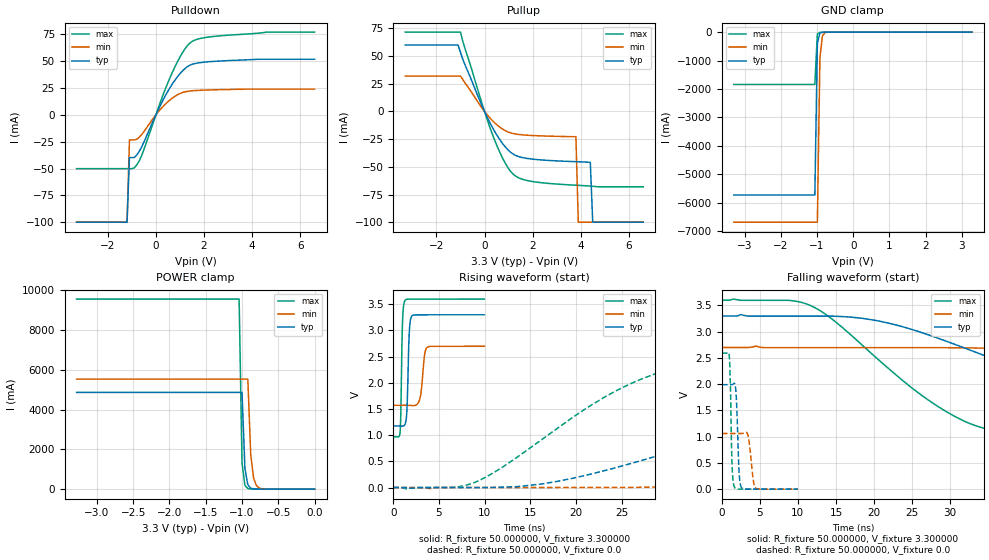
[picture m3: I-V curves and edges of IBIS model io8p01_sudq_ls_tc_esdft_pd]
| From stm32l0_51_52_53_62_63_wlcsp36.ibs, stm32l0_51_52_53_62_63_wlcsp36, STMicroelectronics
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|   Model io8p01_sudq_ls_tc_esdft_pd
[Model]  io8p01_sudq_ls_tc_esdft_pd
Model_type I/O
Polarity   Non-Inverting
Enable   Active-Low
Vinl =   0.990000V
Vinh =   2.310000V
Vmeas =  1.650000V
Cref =   50.000000pF
Rref =   100.000000M
Vref =   0.0V
C_comp   2.248300pF   2.207300pF   2.311900pF
[Temperature Range]   25.000000   0.125000k   -40.000000
[Pullup Reference]   3.300000V   2.700000V   3.600000V
[Pulldown Reference]   0.0V   0.0V   0.0V
[POWER Clamp Reference]   3.300000V   2.700000V   3.600000V
[GND Clamp Reference]   0.0V   0.0V   0.0V
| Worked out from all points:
|   slope of the pulldown table from 0 to 0.495 V, typ, clamps not added: 22.6 ohm
|   slope of the pullup table from 0 to 0.495 V, typ, clamps not added: 23.9 ohm
|   GND clamp passes 1 mA (typ) near -0.64 V on its own axis
|   POWER clamp passes 1 mA (typ) near -0.63 V on its own axis
|   rising waveform, R_fixture 50.000000, V_fixture 3.300000: 20-80 % time 209ps typ, 363ps min, 164ps max; typ from 1.18 V to 3.3 V
|   rising waveform, R_fixture 50.000000, V_fixture 0.0: 20-80 % time 27.9ns typ, 60.5ns min, 14.1ns max; typ from 0 V to 1.99 V
|   falling waveform, R_fixture 50.000000, V_fixture 3.300000: 20-80 % time 24.5ns typ, 54.1ns min, 13.4ns max; typ from 3.3 V to 1.18 V
|   falling waveform, R_fixture 50.000000, V_fixture 0.0: 20-80 % time 290ps typ, 460ps min, 227ps max; typ from 1.99 V to 0 V
[Pulldown]
|Voltage   I(typ)   I(min)   I(max)
-3.3V     -100mA     -100mA     -50.11mA
-1.2V     -100mA     -100mA     -50.11mA
-1.1V     -39.8mA    -23.38mA   -50.11mA
-900mV    -39.8mA    -23.38mA   -49.43mA
-600mV    -30.26mA   -18.59mA   -38.38mA
500mV     22.11mA    12.28mA    30.06mA
900mV     35.58mA    18.71mA    49.62mA
1.3V      44.74mA    21.88mA    64.23mA
1.7V      48.13mA    22.72mA    70.3mA
2.4V      49.79mA    23.3mA     73.03mA
4.6V      51.8mA     24mA       77.1mA
6.6V      51.8mA     24mA       77.1mA
[Pullup]
|Voltage   I(typ)   I(min)   I(max)
-3.3V     60mA       32mA       71.7mA
-1.1V     60mA       32mA       71.7mA
-1V       53.5mA     32mA       71.7mA
-100mV    4.893mA    2.926mA    6.861mA
400mV     -17.21mA   -9.813mA   -24.69mA
900mV     -32.92mA   -17.72mA   -48.15mA
1.3V      -39.75mA   -20.41mA   -58.47mA
3.8V      -45.36mA   -22.8mA    -66.6mA
3.9V      -45.44mA   -100mA     -66.72mA
4.4V      -46mA      -100mA     -67.4mA
4.5V      -100mA     -100mA     -67.56mA
6.6V      -100mA     -100mA     -68mA
[GND_clamp]
|Voltage   I(typ)   I(min)   I(max)
-3.3V     -5.732A    -6.689A    -1.842A
-1.06V    -5.732A    -6.689A    -1.842A
-990mV    -389.4mA   -6.689A    -68.35mA
-920mV    -32.58mA   -918.2mA   -10.73mA
-850mV    -6.776mA   -131mA     -6.518mA
-780mV    -3.484mA   -21.02mA   -4.216mA
3.28V     74.9uA     89.13uA    52.44uA
[POWER_clamp]
|Voltage   I(typ)   I(min)   I(max)
-3.28V    4.87A      5.538A     9.569A
-1.04V    4.87A      5.538A     9.569A
-1V       4.87A      5.538A     1.315A
-960mV    1.032A     5.538A     186.5mA
-920mV    222.2mA    5.538A     31.64mA
-880mV    50.73mA    1.734A     9.582mA
-840mV    13.93mA    544.8mA    5.668mA
-800mV    5.556mA    172.7mA    4.276mA
-760mV    3.231mA    55.84mA    3.297mA
-680mV    1.597mA    6.983mA    1.741mA
0V        0A         0A         0A
[Ramp]
| variable   typ   min   max
dV/dt_r  1.19406/27.83405n   0.63414/60.59668n   1.55520/14.12086n
dV/dt_f  1.27368/24.48233n   0.67122/54.06131n   1.57761/13.39065n
R_load = 50.000000
[Rising Waveform]
R_fixture= 50.000000
V_fixture= 3.300000
V_fixture_min= 2.700000
V_fixture_max= 3.600000
|time   V(typ)   V(min)   V(max)
0s        1.176V     1.571V     970mV
760.8ps   1.175V     1.571V     1.085V
1.021ns   1.172V     1.571V     3.191V
1.281ns   1.207V     1.571V     3.571V
1.502ns   1.515V     1.571V     3.595V
1.782ns   3.042V     1.569V     3.598V
2.042ns   3.277V     1.566V     3.598V
2.923ns   3.298V     1.703V     3.599V
3.744ns   3.299V     2.682V     3.599V
9.97ns    3.299V     2.698V     3.599V
[Rising Waveform]
R_fixture= 50.000000
V_fixture= 0.0
V_fixture_min= 0.0
V_fixture_max= 0.0
|time   V(typ)   V(min)   V(max)
0s        -274.1nV   -2.145uV   54.69nV
8.509ns   -347uV     -126.1uV   70.72mV
16.52ns   75.13mV    -117.3uV   948.2mV
26.53ns   483.2mV    3.851mV    2.025V
33.03ns   825.8mV    16.89mV    2.372V
41.54ns   1.228V     63.78mV    2.525V
57.56ns   1.701V     219.6mV    2.581V
79.58ns   1.923V     502.4mV    2.591V
143.1ns   1.989V     962.4mV    2.592V
249.2ns   1.99V      1.06V      2.592V
[Falling Waveform]
R_fixture= 50.000000
V_fixture= 3.300000
V_fixture_min= 2.700000
V_fixture_max= 3.600000
|time   V(typ)   V(min)   V(max)
0s        3.299V     2.698V     3.599V
11.51ns   3.296V     2.695V     3.507V
20.52ns   3.206V     2.695V     2.473V
29.03ns   2.843V     2.695V     1.519V
33.53ns   2.6V       2.688V     1.201V
39.04ns   2.291V     2.668V     1.064V
54.55ns   1.541V     2.543V     991.9mV
72.07ns   1.285V     2.315V     975.7mV
131.1ns   1.184V     1.709V     970.1mV
249.2ns   1.176V     1.571V     970mV
[Falling Waveform]
R_fixture= 50.000000
V_fixture= 0.0
V_fixture_min= 0.0
V_fixture_max= 0.0
|time   V(typ)   V(min)   V(max)
0s        1.99V      1.06V      2.592V
961ps     1.99V      1.06V      2.545V
1.341ns   1.991V     1.06V      447.1mV
1.662ns   2.014V     1.06V      35.96mV
1.902ns   1.721V     1.06V      5.614mV
2.262ns   320.8mV    1.06V      229.4uV
2.543ns   40.09mV    1.06V      -55.05uV
3.443ns   62.21uV    1.014V     -56.02uV
4.444ns   -14.22uV   21.91mV    -45.39uV
9.97ns    -274.1nV   -2.145uV   54.69nV
